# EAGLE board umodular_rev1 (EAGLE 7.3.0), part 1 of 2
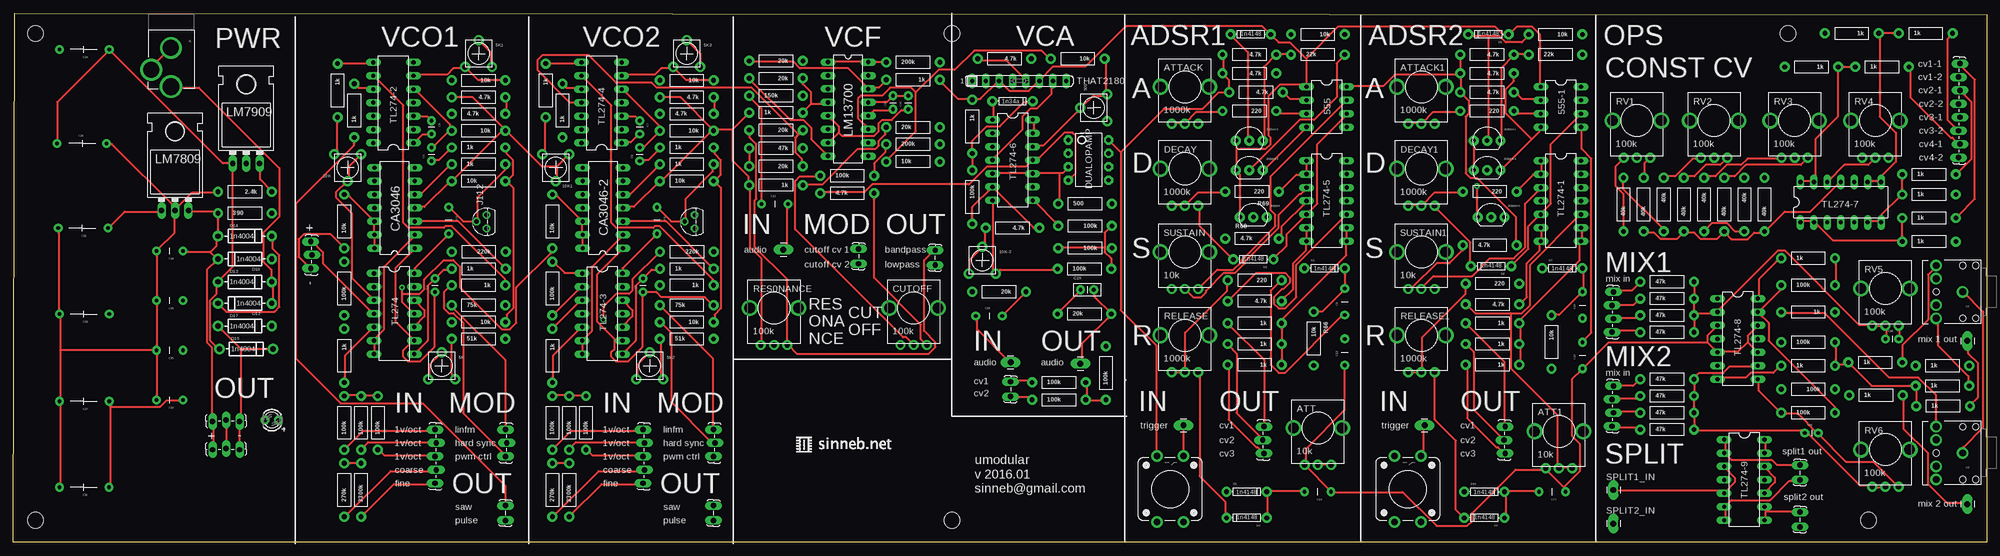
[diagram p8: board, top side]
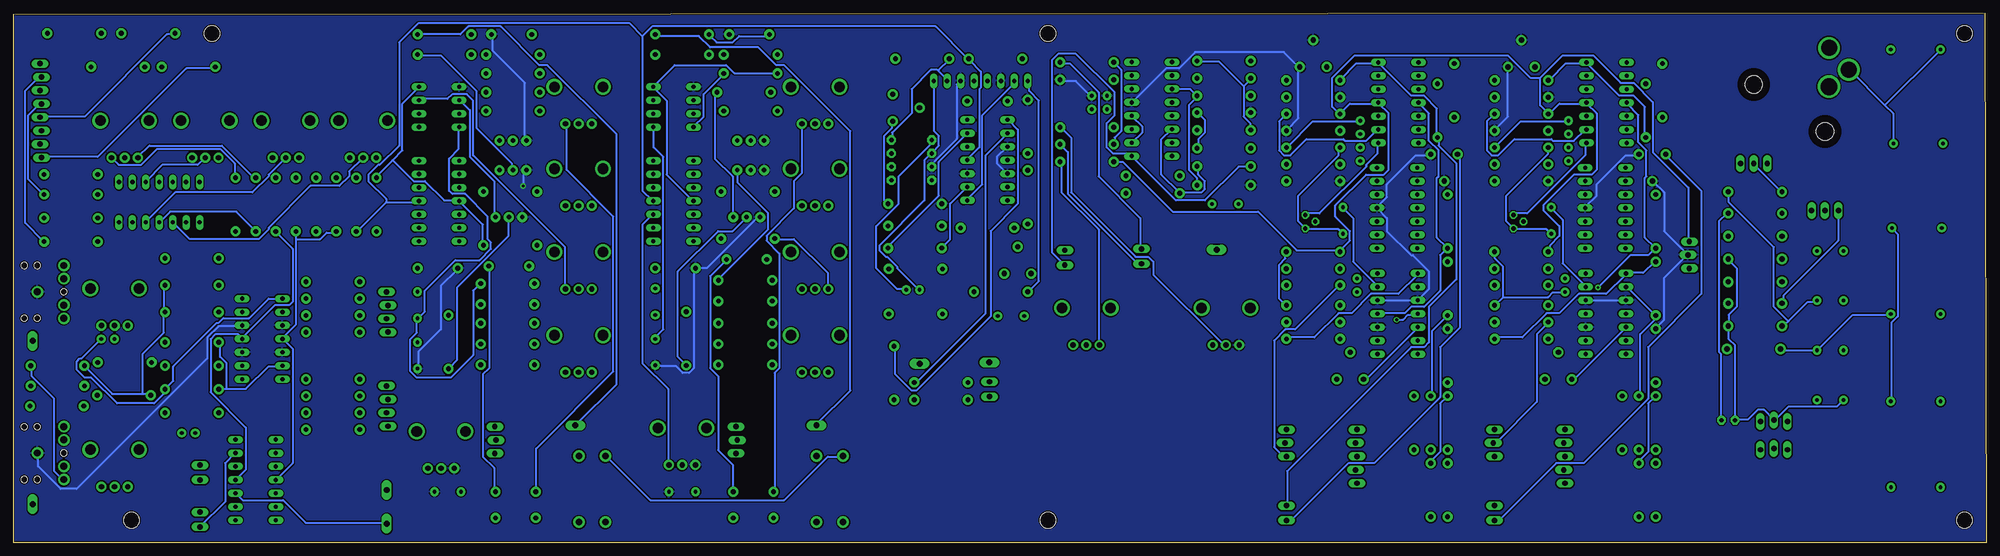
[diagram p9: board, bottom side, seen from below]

Size 373.25 x 100.08 mm. Coordinates in mm from the lower left corner, seen from the top.
Outline: 0,0 0.25,100.08 373.25,99.82 373.25,0 0,0
Copper layers (1*16): Top 0.035mm / dielectric 1.5mm / Bottom 0.035mm
Design rules "SparkFun": minimum track width 8mil, minimum drill 20mil, track to track 8mil, track to pad 8mil, pad to pad 8mil, via to via 8mil, smd to smd 8mil, copper to edge 10mil, drill to drill 8mil, minimum pad ring 12mil, minimum via ring 10mil, stop-mask expansion 4mil, vias tented up to drill 25mil, thermal gap 10mil
Net classes: 0 default: width 0.356 mm, clearance 0.254 mm
Holes 3 mm at 4.19,96.27 4.19,4.19 177.55,4.19 350.9,4.19 335.66,96.27 177.55,96.27

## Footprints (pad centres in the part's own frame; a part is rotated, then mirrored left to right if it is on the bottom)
TO-92-AMMO = drill 0.813 pad 1.88: 1 -2.54,0; 2 0,0; 3 2.54,0
TRIM_POT_PTH = drill 1 pad 1.88: 1 -2.54,-2.54; 2 0,2.54; 3 2.54,-2.54
DIL-08 = drill 0.813 long: 1 -3.81,-3.81; 2 -1.27,-3.81; 3 1.27,-3.81; 4 3.81,-3.81; 5 3.81,3.81; 6 1.27,3.81; 7 -1.27,3.81; 8 -3.81,3.81
ALPS_POT_KIT = drill 1 pad 1.88: P$1 7,-2.5; P$2 7,0; P$3 7,2.5 | drill 2: P$4 0,-4.6; P$5 0,4.6
1X01_LONGPAD = drill 1.118 pad 1.88 long: 1 0,0
CAP-PTH-SMALL = drill 0.7 pad 1.651: 1 0,0; 2 2.54,0
CAP-PTH-5MM = drill 0.7 pad 1.651: 1 -2.5,0; 2 2.5,0
CAP-PTH-SMALL2 = drill 0.7 pad 1.651: 1 0,0; 2 2.54,0
CAP-PTH-LARGE = drill 0.7 pad 1.651: 1 -4.826,0; 2 4.572,0
DIL14 = drill 0.813 long: 1 -7.62,-3.81; 2 -5.08,-3.81; 3 -2.54,-3.81; 4 0,-3.81; 5 2.54,-3.81; 6 5.08,-3.81; 7 7.62,-3.81; 8 7.62,3.81; 9 5.08,3.81; 10 2.54,3.81; 11 0,3.81; 12 -2.54,3.81; 13 -5.08,3.81; 14 -7.62,3.81
1X05_LOCK_LONGPADS = drill 1.016 long: 1 0,0; 2 2.54,-0.254; 3 5.08,0; 4 7.62,-0.254; 5 10.16,0
DIODE-1N4148 = drill 0.9 pad 1.88: A -3.81,0; C 3.81,0
DIODE-1N4001 = drill 1 pad 1.981: A -5.08,0; C 5.08,0
DIP08 = drill 0.813 pad 1.727 octagon: 1 -3.81,-3.81; 2 -1.27,-3.81; 3 1.27,-3.81; 4 3.81,-3.81; 5 3.81,3.81; 6 1.27,3.81; 7 -1.27,3.81; 8 -3.81,3.81
POWER_JACK_PTH_LOCK = drill 2.997 pad 4.115: GND 0.025,6.557; GNDBREAK 3.762,10.7 | drill 3.2 pad 4.115: PWR 0,13.878
TO92 = drill 0.813 octagon: 1 1.27,0; 2 0,1.905; 3 -1.27,0
1X03_LOCK_LONGPADS = drill 1.016 long: 1 0,0; 2 2.54,-0.254; 3 5.08,0
1X02_LOCK_LONGPADS = drill 1.016 long: 1 -0.127,0; 2 2.667,0
1X08_LOCK_LONGPADS = drill 1.016 long: 1 0,0.127; 2 2.54,-0.127; 3 5.08,0.127; 4 7.62,-0.127; 5 10.16,0.127; 6 12.7,-0.127; 7 15.24,0.127; 8 17.78,-0.127
1X04_LOCK_LONGPADS = drill 1.016 long: 1 0,0; 2 2.54,-0.254; 3 5.08,0; 4 7.62,-0.254
LED3MM = drill 0.813 pad 1.676 octagon: A -1.27,0; K 1.27,0
TO-220-ALT = drill 1.016 long: GND 0,-3.81; IN -2.54,-3.81; OUT 2.54,-3.81 | hole 3.302: 0,11.176
DIL16 = drill 0.813 long: 1 -8.89,-3.81; 2 -6.35,-3.81; 3 -3.81,-3.81; 4 -1.27,-3.81; 5 1.27,-3.81; 6 3.81,-3.81; 7 6.35,-3.81; 8 8.89,-3.81; 9 8.89,3.81; 10 6.35,3.81; 11 3.81,3.81; 12 1.27,3.81; 13 -1.27,3.81; 14 -3.81,3.81; 15 -6.35,3.81; 16 -8.89,3.81
AXIAL-0.4 = drill 0.9 pad 1.88: P$1 -5.08,0; P$2 5.08,0
TACTILE-PTH-12MM = drill 1.2 pad 2.159: 1 6.25,-2.5; 2 -6.25,-2.5; 3 6.25,2.5; 4 -6.25,2.5
SIL8 = drill 0.813 long: 1 -8.89,0; 2 -6.35,0; 3 -3.81,0; 4 -1.27,0; 5 1.27,0; 6 3.81,0; 7 6.35,0; 8 8.89,0
AUDIO-JACK = drill 1.3 pad 2.184: RING 5,5; RSH 5,2.5; SLEEVE 0,0; TIP 5,-5; TSH 5,-2.5 | hole 1.2: 0,5; -2.5,5; -2.5,-5; 0,-5; 5,0

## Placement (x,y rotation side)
2N3904  2N3904  [TO-92-AMMO]  234.55,61.52 0 top
2N3904-1  2N3904  [TO-92-AMMO]  278.74,76 0 top
2N3904-2  2N3904  [TO-92-AMMO]  233.79,70.41 0 top
2N3904-3  2N3904  [TO-92-AMMO]  233.79,76 0 top
2N3904-4  2N3904  [TO-92-AMMO]  278.74,70.41 0 top
2N3904-5  2N3904  [TO-92-AMMO]  279.51,61.52 0 top
5K  TRIMPOTPTH  [TRIM_POT_PTH]  81.03,33.4 0 top
5K1  TRIMPOTPTH  [TRIM_POT_PTH]  88.01,92.46 0 top
5K2  TRIMPOTPTH  [TRIM_POT_PTH]  120.4,33.4 0 top
5K3  TRIMPOTPTH  [TRIM_POT_PTH]  127.38,92.46 0 top
10K  TRIMPOTPTH  [TRIM_POT_PTH]  63.25,70.87 180 top
10K1  TRIMPOTPTH  [TRIM_POT_PTH]  102.62,70.87 180 top
10K-2  TRIMPOTPTH  [TRIM_POT_PTH]  183.29,53.37 0 top
500  TRIMPOTPTH  [TRIM_POT_PTH]  204.37,82.2 90 top
555  555  [DIL-08]  248.39,82.35 270 top
555-1  555  [DIL-08]  292.71,82.35 270 top
ATT  10k  [ALPS_POT_KIT]  246.74,21.64 270 top
ATT1  10k  [ALPS_POT_KIT]  292.33,21 270 top
ATTACK  1000k  [ALPS_POT_KIT]  221.59,86.16 270 top
ATTACK1  1000k  [ALPS_POT_KIT]  266.32,86.16 270 top
AUDIO_IN  M01PTH_LONGPAD  [1X01_LONGPAD]  188.62,34.06 90 top
AUDIO_OUT  M01PTH_LONGPAD  [1X01_LONGPAD]  201.83,33.81 90 top
C1  100pF  [CAP-PTH-SMALL]  79.76,47.37 90 top
C2  22nF  [CAP-PTH-5MM]  82.36,60.88 270 top
C3  1nF  [CAP-PTH-SMALL]  79.12,79.76 270 top
C4  10uF  [CAP-PTH-SMALL]  79.12,72.14 90 top
C5  100pF  [CAP-PTH-SMALL]  119.13,47.37 90 top
C6  22nF  [CAP-PTH-5MM]  121.73,60.88 270 top
C7  1nF  [CAP-PTH-SMALL]  118.49,79.76 270 top
C8  10uF  [CAP-PTH-SMALL]  118.49,72.14 90 top
C9  10uF  [CAP-PTH-5MM]  251.82,45.52 90 top
C10  560nF  [CAP-PTH-SMALL]  169.29,81.91 90 top
C11  560nF  [CAP-PTH-SMALL]  166.37,81.91 90 top
C12  1uF  [CAP-PTH-5MM]  144.02,64.01 0 top
C13  10uF  [CAP-PTH-5MM]  251.82,35.99 90 top
C14  2.2uF  [CAP-PTH-5MM]  246.74,9.57 180 top
C15  10uF  [CAP-PTH-5MM]  296.78,44.88 90 top
C16  10uF  [CAP-PTH-5MM]  296.78,35.36 90 top
C17  2.2uF  [CAP-PTH-5MM]  291.06,9.57 180 top
C18  10uf  [CAP-PTH-5MM]  184.56,42.83 0 top
C19  22p  [CAP-PTH-SMALL2]  201.83,47.78 0 top
C20  3300uf  [CAP-PTH-LARGE]  13.31,10.44 180 top
C21  3300uf  [CAP-PTH-LARGE]  13.08,59.44 180 top
C22  1uf  [CAP-PTH-5MM]  29.59,26.92 180 top
C23  3300uf  [CAP-PTH-LARGE]  13.34,43.18 180 top
C24  3300uf  [CAP-PTH-LARGE]  13.34,93.22 180 top
C25  1uf  [CAP-PTH-5MM]  29.59,36.32 180 top
C26  3300uf  [CAP-PTH-LARGE]  13.08,75.44 0 top
C27  3300uf  [CAP-PTH-LARGE]  13.34,26.67 180 top
C28  1uf  [CAP-PTH-5MM]  29.59,55.12 180 top
C29  1uf  [CAP-PTH-5MM]  29.59,45.72 180 top
C30  47pF  [CAP-PTH-SMALL]  354.08,38.48 0 top
C31  47pF  [CAP-PTH-SMALL]  338.84,20.7 0 top
CA3046  CA3046  [DIL14]  72.14,63.25 90 top
CA3046-2  CA3046  [DIL14]  111.51,63.25 90 top
CUTOFF  100k  [ALPS_POT_KIT]  170.31,44.32 270 top
CVS  [1X05_LOCK_LONGPADS]  79.76,11.18 90 top
CVS1  [1X05_LOCK_LONGPADS]  119.13,11.18 90 top
D1  1n4148  [DIODE-1N4148]  234.04,96.06 180 top
D2  1n4148  [DIODE-1N4148]  248.01,51.87 0 top
D3  1n4148  [DIODE-1N4148]  234.55,53.52 180 top
D4  1n4148  [DIODE-1N4148]  233.28,4.62 180 top
D5  1n4148  [DIODE-1N4148]  233.28,9.57 0 top
D6  1n4148  [DIODE-1N4148]  279,96.06 180 top
D7  1n4148  [DIODE-1N4148]  292.97,51.87 0 top
D8  1n4148  [DIODE-1N4148]  279.51,52.25 180 top
D9  1n4148  [DIODE-1N4148]  278.24,4.62 180 top
D10  1n4148  [DIODE-1N4148]  278.24,9.57 0 top
D11  1n34a  [DIODE-1N4148]  189,83.47 0 top
D12  1n4004  [DIODE-1N4001]  43.82,45.21 180 top
D13  1n4004  [DIODE-1N4001]  43.82,49.28 0 top
D14  1n4004  [DIODE-1N4001]  43.82,57.91 0 top
D15  1n4004  [DIODE-1N4001]  44.07,36.58 0 top
D16  1n4004  [DIODE-1N4001]  43.82,53.59 180 top
D17  1n4004  [DIODE-1N4001]  43.82,40.89 0 top
DECAY  1000k  [ALPS_POT_KIT]  221.59,70.66 270 top
DECAY1  1000k  [ALPS_POT_KIT]  266.32,70.66 270 top
DUALOPAMP  OPAMP-DUALDIP  [DIP08]  203.35,72.29 270 top
J1  POWER_JACKPTH_LOCK  [POWER_JACK_PTH_LOCK]  29.84,100.08 180 top
J112  J201  [TO92]  89.52,60.66 90 top
JP1  [1X03_LOCK_LONGPADS]  93.09,16.26 90 top
JP2  [1X02_LOCK_LONGPADS]  93.07,4.29 90 top
JP3  [1X03_LOCK_LONGPADS]  56.26,51.82 90 top
JP4  [1X03_LOCK_LONGPADS]  132.46,16.26 90 top
JP5  [1X02_LOCK_LONGPADS]  132.44,4.29 90 top
JP6  M01PTH_LONGPAD  [1X01_LONGPAD]  145.67,55.37 90 top
JP7  FLT_OUT  [1X02_LOCK_LONGPADS]  174.37,55.12 270 top
JP8  CV_IN  [1X02_LOCK_LONGPADS]  159.89,52.83 90 top
JP9  CV_OUT  [1X03_LOCK_LONGPADS]  236.58,21.89 270 top
JP10  CV_OUT  [1X03_LOCK_LONGPADS]  282.17,21.89 270 top
JP11  cv_in  [1X02_LOCK_LONGPADS]  188.62,27.71 90 top
JP12  pwr_out_1  [1X03_LOCK_LONGPADS]  42.8,22.86 180 top
JP13  pwr_out_2  [1X03_LOCK_LONGPADS]  42.8,17.53 180 top
JP14  [1X08_LOCK_LONGPADS]  368.05,90.55 270 top
JP15  [1X04_LOCK_LONGPADS]  302.64,47.37 270 top
JP16  [1X04_LOCK_LONGPADS]  302.64,29.59 270 top
JP17  split2_out  [1X02_LOCK_LONGPADS]  337.95,5.59 270 top
JP18  split1_out  [1X02_LOCK_LONGPADS]  337.95,14.48 270 top
JP19  M01PTH_LONGPAD  [1X01_LONGPAD]  369.57,38.1 0 top
JP20  M01PTH_LONGPAD  [1X01_LONGPAD]  369.57,7.24 0 top
LED1  green  [LED3MM]  48.9,23.11 180 top
LM7809  LM7809  [TO-220-ALT]  30.61,66.55 0 top
LM7909  LM7909  [TO-220-ALT]  44.07,75.44 0 top
LM13700  LM13700N  [DIL16]  157.9,81.94 270 top
Q2  J201  [TO92]  128.89,60.66 90 top
R1  100k  [AXIAL-0.4]  62.61,48.01 90 top
R2  100k  [AXIAL-0.4]  62.61,22.61 90 top
R3  100k  [AXIAL-0.4]  65.79,22.61 90 top
R4  100k  [AXIAL-0.4]  68.96,22.61 90 top
R5  270k  [AXIAL-0.4]  62.61,9.91 90 top
R6  3300k  [AXIAL-0.4]  65.79,9.91 90 top
R7  51k  [AXIAL-0.4]  88.01,38.48 0 top
R8  1k  [AXIAL-0.4]  62.61,35.31 270 top
R9  220k  [AXIAL-0.4]  88.03,54.98 180 top
R10  1k  [AXIAL-0.4]  88.03,51.73 0 top
R11  75k  [AXIAL-0.4]  88.01,44.83 0 top
R12  1k  [AXIAL-0.4]  88.01,71.5 0 top
R13  1k  [AXIAL-0.4]  88.01,74.68 0 top
R14  4.7k  [AXIAL-0.4]  88.01,81.03 0 top
R15  4.7k  [AXIAL-0.4]  88.01,84.2 180 top
R16  10k  [AXIAL-0.4]  88.01,41.66 180 top
R17  10k  [AXIAL-0.4]  88.01,68.33 0 top
R18  10k  [AXIAL-0.4]  88.01,77.85 180 top
R19  10k  [AXIAL-0.4]  88.01,87.38 180 top
R20  1k  [AXIAL-0.4]  64.52,81.66 90 top
R21  1k  [AXIAL-0.4]  88.01,48.64 180 top
R22  1k  [AXIAL-0.4]  61.34,85.47 270 top
R23  10k  [AXIAL-0.4]  62.61,60.71 90 top
R24  100k  [AXIAL-0.4]  101.98,48.01 90 top
R25  100k  [AXIAL-0.4]  101.98,22.61 90 top
R26  100k  [AXIAL-0.4]  105.16,22.61 90 top
R27  100k  [AXIAL-0.4]  108.33,22.61 90 top
R28  270k  [AXIAL-0.4]  101.98,9.91 90 top
R29  3300k  [AXIAL-0.4]  105.16,9.91 90 top
R30  51k  [AXIAL-0.4]  127.38,38.48 0 top
R31  1k  [AXIAL-0.4]  101.98,35.31 270 top
R32  220k  [AXIAL-0.4]  127.4,54.98 180 top
R33  1k  [AXIAL-0.4]  127.4,51.73 0 top
R34  75k  [AXIAL-0.4]  127.38,44.83 0 top
R35  1k  [AXIAL-0.4]  127.38,71.5 0 top
R36  1k  [AXIAL-0.4]  127.38,74.68 0 top
R37  4.7k  [AXIAL-0.4]  127.38,81.03 0 top
R38  4.7k  [AXIAL-0.4]  127.38,84.2 180 top
R39  10k  [AXIAL-0.4]  127.38,41.66 180 top
R40  10k  [AXIAL-0.4]  127.38,68.33 0 top
R41  10k  [AXIAL-0.4]  127.38,77.85 180 top
R42  10k  [AXIAL-0.4]  127.38,87.38 180 top
R43  1k  [AXIAL-0.4]  103.89,81.66 90 top
R44  1k  [AXIAL-0.4]  127.38,48.64 180 top
R45  1k  [AXIAL-0.4]  100.71,85.47 270 top
R46  10k  [AXIAL-0.4]  101.98,60.71 90 top
R47  150k  [AXIAL-0.4]  144.27,84.45 0 top
R48  1k  [AXIAL-0.4]  144.27,67.56 180 top
R49  20k  [AXIAL-0.4]  144.27,91.06 180 top
R50  20k  [AXIAL-0.4]  144.27,77.98 180 top
R51  20k  [AXIAL-0.4]  144.27,87.76 180 top
R52  20k  [AXIAL-0.4]  144.27,71.12 180 top
R53  47k  [AXIAL-0.4]  144.27,74.55 180 top
R54  20k  [AXIAL-0.4]  170.18,78.49 0 top
R55  1k  [AXIAL-0.4]  144.27,81.28 0 top
R56  1k  [AXIAL-0.4]  170.18,87.5 180 top
R57  200k  [AXIAL-0.4]  170.18,90.8 0 top
R58  200k  [AXIAL-0.4]  170.18,75.31 0 top
R59  4.7k  [AXIAL-0.4]  157.73,66.04 0 top
R60  10k  [AXIAL-0.4]  170.18,72.01 0 top
R61  100k  [AXIAL-0.4]  157.73,69.34 0 top
R62  10k  [AXIAL-0.4]  246.74,96.06 180 top
R63  4.7k  [AXIAL-0.4]  233.79,92.25 180 top
R64  22k  [AXIAL-0.4]  246.74,92.25 0 top
R65  4.7k  [AXIAL-0.4]  233.79,88.7 180 top
R66  10k  [AXIAL-0.4]  245.98,38.53 270 top
R67  4.7k  [AXIAL-0.4]  235.06,85.14 180 top
R68  4.7k  [AXIAL-0.4]  234.29,57.45 0 top
R69  220  [AXIAL-0.4]  234.29,66.34 180 top
R70  220  [AXIAL-0.4]  234.8,49.58 180 top
R71  220  [AXIAL-0.4]  233.79,81.58 180 top
R72  4.7k  [AXIAL-0.4]  234.8,45.64 180 top
R73  1k  [AXIAL-0.4]  234.8,41.45 180 top
R74  1k  [AXIAL-0.4]  234.8,37.51 180 top
R75  1k  [AXIAL-0.4]  234.8,33.58 180 top
R76  10k  [AXIAL-0.4]  291.7,96.06 180 top
R77  4.7k  [AXIAL-0.4]  278.74,92.25 180 top
R78  22k  [AXIAL-0.4]  291.7,92.25 0 top
R79  4.7k  [AXIAL-0.4]  278.74,88.7 180 top
R80  10k  [AXIAL-0.4]  290.94,37.9 270 top
R81  4.7k  [AXIAL-0.4]  278.74,85.14 180 top
R82  4.7k  [AXIAL-0.4]  279.25,56.18 0 top
R83  220  [AXIAL-0.4]  279.25,66.34 180 top
R84  220  [AXIAL-0.4]  279.76,48.94 180 top
R85  220  [AXIAL-0.4]  278.74,81.58 180 top
R86  4.7k  [AXIAL-0.4]  279.76,45.01 180 top
R87  1k  [AXIAL-0.4]  279.76,41.45 180 top
R88  1k  [AXIAL-0.4]  279.76,37.51 180 top
R89  1k  [AXIAL-0.4]  279.76,33.58 180 top
R90  100k  [AXIAL-0.4]  206.66,32.03 90 top
R91  100k  [AXIAL-0.4]  197.77,30.25 0 top
R92  100k  [AXIAL-0.4]  197.77,26.95 0 top
R93  1k  [AXIAL-0.4]  181.38,78.64 270 top
R94  100k  [AXIAL-0.4]  181.38,65.31 270 top
R95  4.7k  [AXIAL-0.4]  189,59.46 180 top
R96  100k  [AXIAL-0.4]  202.59,51.72 0 top
R97  100k  [AXIAL-0.4]  202.72,59.85 180 top
R98  10k  [AXIAL-0.4]  201.32,91.47 180 top
R99  500  [AXIAL-0.4]  202.72,64.04 0 top
R100  100k  [AXIAL-0.4]  202.72,55.65 180 top
R101  4.7k  [AXIAL-0.4]  187.48,91.47 180 top
R102  20k  [AXIAL-0.4]  186.46,47.4 180 top
R103  20k  [AXIAL-0.4]  202.59,43.21 0 top
R104  390  [AXIAL-0.4]  43.82,62.23 0 top
R105  2.4k  [AXIAL-0.4]  43.82,66.29 180 top
R106  1k  [AXIAL-0.4]  362.33,61.34 0 top
R107  1k  [AXIAL-0.4]  362.33,56.9 0 top
R108  1k  [AXIAL-0.4]  362.33,69.6 0 top
R109  1k  [AXIAL-0.4]  362.33,65.79 0 top
R110  1k  [AXIAL-0.4]  347.73,96.27 180 top
R111  1k  [AXIAL-0.4]  361.7,96.27 0 top
R112  1k  [AXIAL-0.4]  353.44,89.92 0 top
R113  1k  [AXIAL-0.4]  340.11,89.92 180 top
R114  40k  [AXIAL-0.4]  304.55,63.88 90 top
R115  47k  [AXIAL-0.4]  312.8,39.75 0 top
R116  47k  [AXIAL-0.4]  312.8,42.93 0 top
R117  47k  [AXIAL-0.4]  312.8,46.1 0 top
R118  100k  [AXIAL-0.4]  339.47,28.96 180 top
R119  100k  [AXIAL-0.4]  339.47,37.85 0 top
R120  1k  [AXIAL-0.4]  339.47,33.4 0 top
R121  40k  [AXIAL-0.4]  308.36,63.88 90 top
R122  40k  [AXIAL-0.4]  312.17,63.88 270 top
R123  40k  [AXIAL-0.4]  319.79,63.88 270 top
R124  40k  [AXIAL-0.4]  327.41,63.88 270 top
R125  40k  [AXIAL-0.4]  331.22,63.88 90 top
R126  40k  [AXIAL-0.4]  323.6,63.88 90 top
R127  40k  [AXIAL-0.4]  315.98,63.88 90 top
R128  1k  [AXIAL-0.4]  352.17,34.04 0 top
R129  1k  [AXIAL-0.4]  364.87,29.59 0 top
R130  47k  [AXIAL-0.4]  312.8,49.28 0 top
R131  47k  [AXIAL-0.4]  312.8,21.34 0 top
R132  47k  [AXIAL-0.4]  312.8,24.51 0 top
R133  47k  [AXIAL-0.4]  312.8,27.69 0 top
R134  100k  [AXIAL-0.4]  339.47,24.51 0 top
R135  100k  [AXIAL-0.4]  339.47,48.64 0 top
R136  1k  [AXIAL-0.4]  339.47,53.72 0 top
R137  1k  [AXIAL-0.4]  339.47,43.56 180 top
R138  1k  [AXIAL-0.4]  364.87,33.4 0 top
R139  47k  [AXIAL-0.4]  312.8,30.86 0 top
R140  1k  [AXIAL-0.4]  365,25.78 0 top
R141  1k  [AXIAL-0.4]  352.3,27.81 0 top
RELEASE  1000k  [ALPS_POT_KIT]  221.59,39.17 270 top
RELEASE1  1000k  [ALPS_POT_KIT]  266.32,39.17 270 top
RES0NANCE  100k  [ALPS_POT_KIT]  143.89,44.32 270 top
RV1  100k  [ALPS_POT_KIT]  307.09,79.76 270 top
RV2  100k  [ALPS_POT_KIT]  321.69,79.76 270 top
RV3  100k  [ALPS_POT_KIT]  336.93,79.76 270 top
RV4  100k  [ALPS_POT_KIT]  352.17,79.76 270 top
RV5  100k  [ALPS_POT_KIT]  354.08,48.01 270 top
RV6  100k  [ALPS_POT_KIT]  354.08,17.53 270 top
S1  SWITCH-MOMENTARY-212MM  [TACTILE-PTH-12MM]  218.8,10.08 90 top
S2  SWITCH-MOMENTARY-212MM  [TACTILE-PTH-12MM]  263.76,10.08 90 top
SPLIT1_IN  M01PTH_LONGPAD  [1X01_LONGPAD]  302.64,9.91 0 top
SPLIT2_IN  M01PTH_LONGPAD  [1X01_LONGPAD]  302.64,3.56 0 top
SUSTAIN  10k  [ALPS_POT_KIT]  221.59,54.91 270 top
SUSTAIN1  10k  [ALPS_POT_KIT]  266.32,54.91 270 top
THAT2180  [SIL8]  190.27,87.28 0 top
TL274  QUAD_OPAMPP  [DIL14]  72.05,43.24 270 top
TL274-1  QUAD_OPAMPP  [DIL14]  292.71,64.57 270 top
TL274-2  QUAD_OPAMPP  [DIL14]  71.9,83.16 90 top
TL274-3  QUAD_OPAMPP  [DIL14]  111.42,43.24 270 top
TL274-4  QUAD_OPAMPP  [DIL14]  111.27,83.16 90 top
TL274-5  QUAD_OPAMPP  [DIL14]  248.39,64.57 270 top
TL274-6  QUAD_OPAMPP  [DIL14]  189,72.29 270 top
TL274-7  QUAD_OPAMPP  [DIL14]  345.63,64.34 0 top
TL274-8  QUAD_OPAMPP  [DIL14]  326.14,38.48 270 top
TL274-9  QUAD_OPAMPP  [DIL14]  327.41,11.81 270 top
TRIG_IN  M01PTH_LONGPAD  [1X01_LONGPAD]  221.34,22.15 90 top
TRIG_IN1  M01PTH_LONGPAD  [1X01_LONGPAD]  266.93,22.15 90 top
U1  [AUDIO-JACK]  368.68,47.37 180 top
U2  [AUDIO-JACK]  368.68,16.89 180 top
